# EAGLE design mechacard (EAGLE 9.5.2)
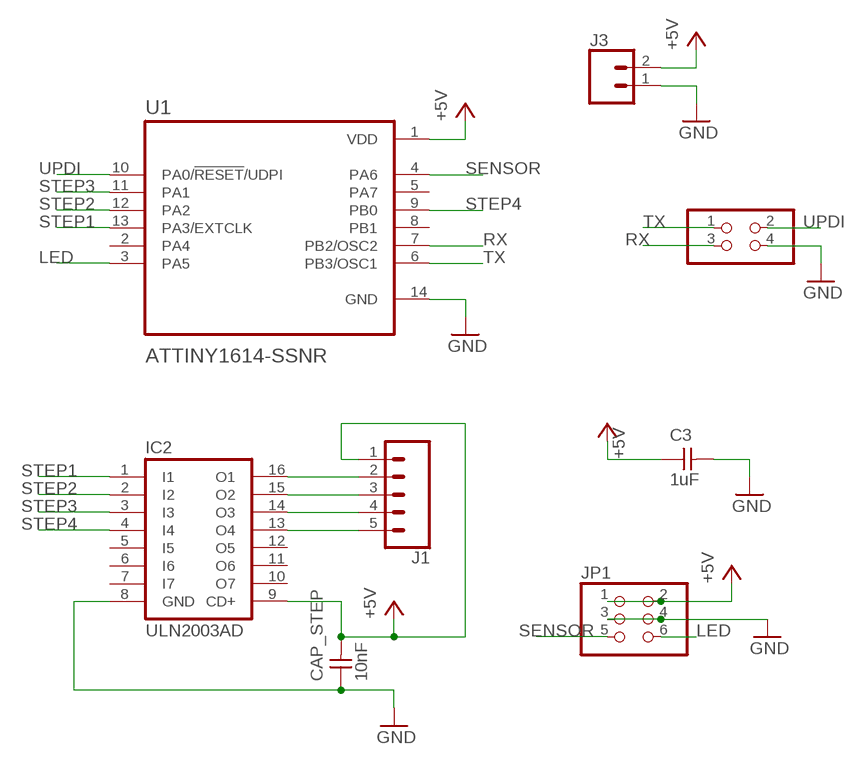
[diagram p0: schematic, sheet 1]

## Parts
C3  1uF  CAP_UNPOLARIZEDFAB  [C1206FAB]
CAP_STEP  10nF  CAP_UNPOLARIZEDFAB  [C1206FAB]
IC2  ULN2003AD  [SO16]
J1  CONN_05JST-VERT  [JST-5-PTH-VERT]
J3  CONN_02  [1X02]
JP1  CONN_03X2-PINHEAD-SMD  [2X03SMD]
U1  ATTINY1614-SSNR  [SOIC127P600X175-14N]
U$1  CONN_02X2-PINHEAD-SMD  [2X02SMD]

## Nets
+5V: C3.1 CAP_STEP.2 IC2.9(CD+) J1.1 J3.2 JP1.1 JP1.2 U1.1(VDD)
GND: C3.2 CAP_STEP.1 IC2.8(GND) J3.1 JP1.3 JP1.4 U1.14(GND) U$1.4
LED: JP1.6 U1.3(PA5)
N$1: IC2.16(O1) J1.2
N$2: IC2.15(O2) J1.3
N$3: IC2.14(O3) J1.4
N$4: IC2.13(O4) J1.5
RX: U1.7(PB2/OSC2) U$1.3
SENSOR: JP1.5 U1.4(PA6)
STEP1: IC2.1(I1) U1.13(PA3/EXTCLK)
STEP2: IC2.2(I2) U1.12(PA2)
STEP3: IC2.3(I3) U1.11(PA1)
STEP4: IC2.4(I4) U1.9(PB0)
TX: U1.6(PB3/OSC1) U$1.1
UPDI: U1.10(PA0/!RESET!/UDPI) U$1.2
Unconnected: IC2.5(I5) IC2.6(I6) IC2.7(I7) IC2.10(O7) IC2.11(O6) IC2.12(O5) U1.2(PA4) U1.5(PA7) U1.8(PB1)

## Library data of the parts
C3 CAP_STEP = eagle_fab:CAP_UNPOLARIZED
IC2 = uln-udn:ULN2003A: DRIVER ARRAY
J1 = SparkFun-Connectors:CONN_05: Multi connection point. Often used as Generic Header-pin footprint for 0.1 inch spaced/style header connections On any of the 0.1 inch spaced packages, you can populate with these: Break Away Headers - Straight (PRT-00116) Break Away Male Headers - Right Angle (PRT-00553) Female Headers (PRT-00115)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
J3 = SparkFun-Connectors:CONN_02: Multi connection point. Often used as Generic Header-pin footprint for 0.1 inch spaced/style header connections
JP1 = eagle_fab:CONN_03X2-PINHEAD-SMD: PIN HEADER
U1 = ATTINY1614-SSNR:ATTINY1614-SSNR: 20MHz, SOIC, 85C, Green, 14 SOIC .150in T/R; AVAILABILITY: Unavailable; DESCRIPTION: AVR tinyAVR™ 1 Microcontroller IC 8-Bit 20MHz 16KB _16K x 8_ FLASH 14-SOIC; MF: Microchip; MP: ATTINY1614-SSNR; PACKAGE: SO-14 Microchip; PRICE: None
U$1 = eagle_fab:CONN_02X2-PINHEAD-SMD

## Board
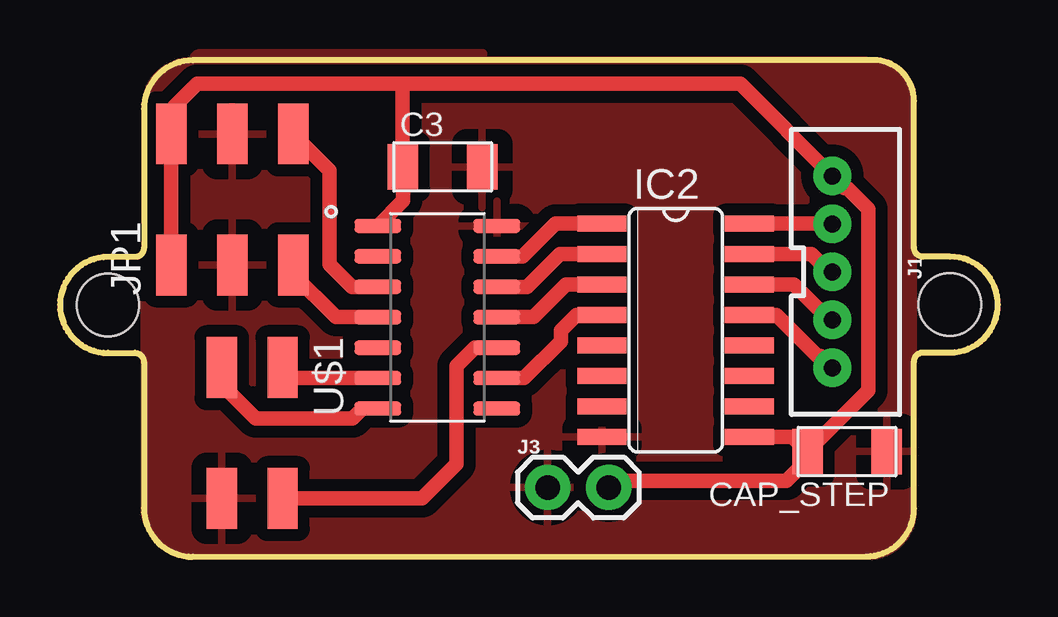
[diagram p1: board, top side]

Size 39.1 x 20.72 mm. Coordinates in mm from the lower left corner, seen from the top.
Outline: 3.12,12.5 2,12.5 arc180 2,8.5 3.12,8.5 arc-95 3.5,8.09 3.5,2.03 arc90 5.53,0 33.6,0.02 arc90 35.6,2.02 35.6,8.14 arc-90 35.98,8.52 37.1,8.52 arc180 37.1,12.52 35.98,12.52 arc-90 35.6,12.9 35.6,19.02 arc90 33.9,20.72 5.53,20.7 arc90 3.5,18.67 3.5,12.88 arc-90 3.12,12.5
Copper layers (1*16): Top 0.035mm / dielectric 1.5mm / Bottom 0.035mm
Design rules "OthermillDRC_1_64_v2 *": minimum track width 16mil, minimum drill 31mil, track to track 0.5mm, track to pad 0.39878125mm, pad to pad 0.39878125mm, via to via 0.39878125mm, smd to smd 0mil, copper to edge 0mil, drill to drill 1mil, minimum pad ring 0mil, minimum via ring 15mil, stop-mask expansion 1mil, vias tented up to drill 30mil, thermal gap 25mil
Holes 2.6 mm at 37.1,10.52 2,10.5

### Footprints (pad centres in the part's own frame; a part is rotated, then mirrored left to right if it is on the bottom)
C1206FAB = smd 1.27 x 1.905: 1 -1.651,0; 2 1.651,0
SO16 = smd 0.66 x 2.032: 1 -4.445,-3.073; 2 -3.175,-3.073; 3 -1.905,-3.073; 4 -0.635,-3.073; 5 0.635,-3.073; 6 1.905,-3.073; 7 3.175,-3.073; 8 4.445,-3.073; 9 4.445,3.073; 10 3.175,3.073; 11 1.905,3.073; 12 0.635,3.073; 13 -0.635,3.073; 14 -1.905,3.073; 15 -3.175,3.073; 16 -4.445,3.073
JST-5-PTH-VERT = drill 0.7 pad 1.6: 1 -4,0.18; 2 -2,0.18; 3 0,0.18; 4 2,0.18; 5 4,0.18
1X02 = drill 1.016 pad 1.88: 1 0,0; 2 2.54,0
2X03SMD = smd 2.54 x 1.27: 1 -2.54,2.54; 2 2.92,2.54; 3 -2.54,0; 4 2.92,0; 5 -2.54,-2.54; 6 2.92,-2.54
SOIC127P600X175-14N = smd 1.95 x 0.59: 1 -2.48,3.81; 2 -2.48,2.54; 3 -2.48,1.27; 4 -2.48,0; 5 -2.48,-1.27; 6 -2.48,-2.54; 7 -2.48,-3.81; 8 2.48,-3.81; 9 2.48,-2.54; 10 2.48,-1.27; 11 2.48,0; 12 2.48,1.27; 13 2.48,2.54; 14 2.48,3.81
2X02SMD = smd 2.54 x 1.27: 1 -2.54,1.27; 2 2.92,1.27; 3 -2.54,-1.27; 4 2.92,-1.27

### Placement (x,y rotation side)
C3  15.95,16.26 0 top
CAP_STEP  32.81,4.39 180 top
IC2  25.67,9.45 270 top
J1  32.02,11.88 270 top
J3  20.33,2.89 0 top
JP1  7.18,14.71 90 top
U1  15.73,9.99 0 top
U$1  8.01,5.35 270 top

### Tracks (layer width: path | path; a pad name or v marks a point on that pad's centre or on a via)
+5V
  Top 0.61: 14.28,19.72 28.36,19.72 J1.1 32.7,15.38 32.82,15.38 33.7,14.5 33.7,6.93 CAP_STEP.2 | U1.1 14.3,14.85 C3.1 14.28,16.27 14.28,19.72 | J3.2 23.14,3.16 30.28,3.16 31.16,4.04 CAP_STEP.2 | IC2.9 30.54,5 CAP_STEP.2 | JP1.1 JP1.2 | JP1.2 4.64,17.89 | 14.28,19.72 5.71,19.72 4.77,18.78 4.77,17.76 JP1.2
GND
  pour Top: 17.66,20.59 arc-90 17.79,20.72 33.41,20.72 arc-90 35.57,18.56 35.57,1.92 arc-90 33.66,0.02 5.64,0.02 arc-90 3.5,2.16 3.5,18.67 arc-90 5.53,20.7 arc-90 5.85,21.02 17.6,21.02 arc-90 17.66,20.95
LED
  Top 0.61: U1.3 12.18,11.26 11.25,12.19 11.25,16.11 JP1.6
N$1
  Top 0.61: IC2.16 32.18,13.89 J1.2
N$2
  Top 0.61: IC2.15 31.33,12.62 32.07,11.88 J1.3
N$3
  Top 0.61: IC2.14 30.6,11.35 31.58,10.37 31.6,10.37 32.09,9.88 J1.4
N$4
  Top 0.61: J1.5 31.7,8.37 31.58,8.37 29.87,10.08 IC2.13
RX
  Top 0.61: U1.7 12.62,6.18 12.21,5.76 8.15,5.76 6.67,7.24 6.67,7.83 U$1.3
SENSOR
  Top 0.61: JP1.5 9.72,11.78 11.51,9.99 U1.4
STEP1
  Top 0.61: U1.13 19.28,12.53 20.65,13.89 IC2.1
STEP2
  Top 0.61: U1.12 19.48,11.26 20.84,12.62 IC2.2
STEP3
  Top 0.61: U1.11 19.73,9.99 21.1,11.35 IC2.3
STEP4
  Top 0.61: U1.9 19.35,7.45 20.88,8.97 20.88,9.44 21.52,10.08 IC2.4
TX
  Top 0.61: U1.6 9.73,7.45 U$1.1
UPDI
  Top 0.61: U$1.2 15.1,2.43 16.53,3.87 16.53,7.95 17.3,8.72 U1.10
